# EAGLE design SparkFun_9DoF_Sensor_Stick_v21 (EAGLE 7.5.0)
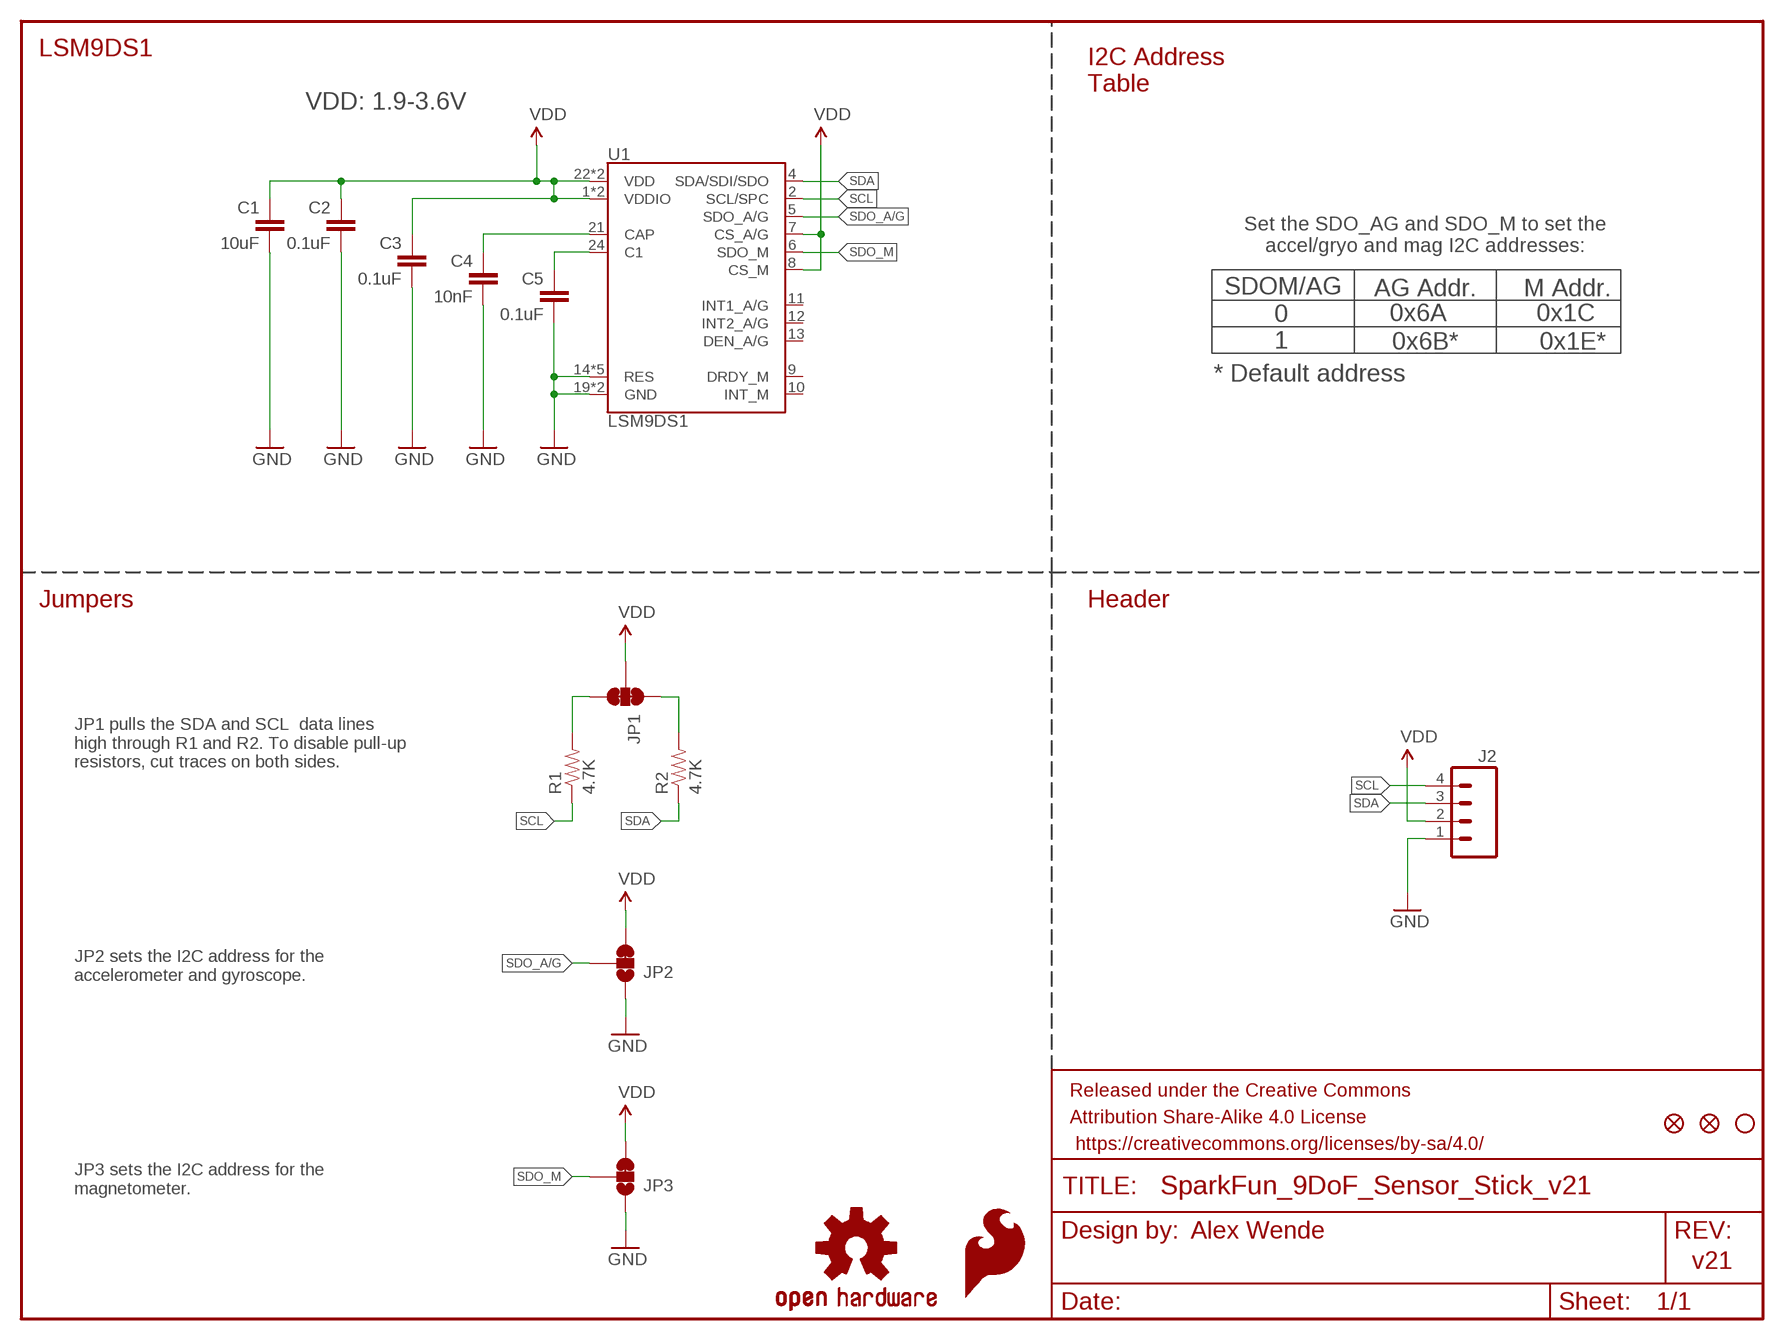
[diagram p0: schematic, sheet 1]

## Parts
C1  10uF  10UF-6.3V-20%(0603)  [0603-CAP]
C2  0.1uF  0.1UF-25V(+80/-20%)(0603)  [0603-CAP]
C3  0.1uF  0.1UF-25V(+80/-20%)(0603)  [0603-CAP]
C4  10nF  10NF/10000PF-50V-10%(0603)  [0603-CAP]
C5  0.1uF  0.1UF-25V(+80/-20%)(0603)  [0603-CAP]
FD3  FIDUCIALUFIDUCIAL  [MICRO-FIDUCIAL]
FD4  FIDUCIALUFIDUCIAL  [MICRO-FIDUCIAL]
FRAME1  FRAME-LETTER  [CREATIVE_COMMONS]
H1  STAND-OFF  [STAND-OFF]
J2  M04NO_SILK_ALL_ROUND  [1X04_NO_SILK_ALL_ROUND]
JP1  JUMPER-PAD-3-NC_BY_TRACE  [PAD-JUMPER-3-3OF3_NC_BY_TRACE_YES_SILK_FULL_BOX]
JP2  JUMPER-PAD-3-2OF3_NC_BY_TRACE_SMALL  [PAD-JUMPER-3-2OF3_NC_BY_TRACE_YES_SILK_FULL_BOX]
JP3  JUMPER-PAD-3-2OF3_NC_BY_TRACE_SMALL  [PAD-JUMPER-3-2OF3_NC_BY_TRACE_YES_SILK_FULL_BOX]
LOGO1  SFE_LOGO_FLAME.1_INCH  [SFE_LOGO_FLAME_.1]
LOGO3  OSHW-LOGOMINI  [OSHW-LOGO-MINI]
R1  4.7K  4.7KOHM-1/10W-1%(0603)  [0603-RES]
R2  4.7K  4.7KOHM-1/10W-1%(0603)  [0603-RES]
U1  LSM9DS1  [LGA24-8X4]

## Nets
GND: C1.2 C2.2 C3.2 C4.2 C5.2 J2.1 JP2.1 JP3.1 U1.14(RES) U1.15(RES) U1.16(RES) U1.17(RES) U1.18(RES) U1.19(GND) U1.20(GND)
N$1: JP1.1 R2.2
N$2: JP1.3 R1.2
N$5: C4.1 U1.21(CAP)
N$6: C5.1 U1.24(C1)
SCL: J2.4 R1.1 U1.2(SCL/SPC)
SDA: J2.3 R2.1 U1.4(SDA/SDI/SDO)
SDO_A/G: JP2.2 U1.5(SDO_A/G)
SDO_M: JP3.2 U1.6(SDO_M)
VDD: C1.1 C2.1 C3.1 J2.2 JP1.2 JP2.3 JP3.3 U1.1(VDDIO) U1.3(VDDIO) U1.7(CS_A/G) U1.8(CS_M) U1.22(VDD) U1.23(VDD)
Unconnected: U1.9(DRDY_M) U1.10(INT_M) U1.11(INT1_A/G) U1.12(INT2_A/G) U1.13(DEN_A/G)

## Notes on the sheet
- LSM9DS1
- I2C Address
  Table
- VDD: 1.9-3.6V
- Set the SDO_AG and SDO_M to set the
  accel/gryo and mag I2C addresses:
- SDOM/AG | AG Addr. | M Addr.
- 0x6A | 0x1C
- 0
  1
- 0x6B* | 0x1E*
- * Default address
- Jumpers | Header
- JP1 pulls the SDA and SCL  data lines
  high through R1 and R2. To disable pull-up
  resistors, cut traces on both sides.
- JP2 sets the I2C address for the
  accelerometer and gyroscope.
- JP3 sets the I2C address for the
  magnetometer.
- Alex Wende
- v21

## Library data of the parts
C1 = SparkFun-Capacitors:10UF-6.3V-20%(0603): CAP-11015; PROD_ID: CAP-11015
C2 C3 C5 = SparkFun-Capacitors:0.1UF-25V(+80/-20%)(0603): CAP-00810; PROD_ID: CAP-00810
C4 = SparkFun-Capacitors:10NF/10000PF-50V-10%(0603): CAP-00867; PROD_ID: CAP-00867
FD3 FD4 = SparkFun-Aesthetics:FIDUCIAL: Fiducial Alignment Points
FRAME1 = SparkFun-Aesthetics:FRAME-LETTER: Schematic Frame
H1 = SparkFun-Electromechanical:STAND-OFF: #4 Stand Off
J2 = SparkFun-Connectors:M04: Header 4 Standard 4-pin 0.1" header. Use with straight break away headers (SKU : PRT-00116), right angle break away headers (PRT-00553), swiss pins (PRT-00743), machine pins (PRT-00117), and female headers (PRT-00115). Molex polarized connector foot print use with SKU : PRT-08231 with associated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; PROD_ID: CONN-09696
JP1 = SparkFun-Passives:JUMPER-PAD-3-NC_BY_TRACE
JP2 JP3 = SparkFun-Passives:JUMPER-PAD-3-2OF3_NC_BY_TRACE
LOGO1 = SparkFun-Aesthetics:SFE_LOGO_FLAME: SFE Logo, flame only
LOGO3 = SparkFun-Aesthetics:OSHW-LOGO: Open Source Hardware Logo
R1 R2 = SparkFun-Resistors:4.7KOHM-1/10W-1%(0603): RES-07857; PROD_ID: RES-07857
U1 = SparkFun-Sensors:LSM9DS1: LSM9DS1 3D accelerometer, gyroscope & magnetometer The LSM9DS1 is a system-in-package featuring a 3D digital linear acceleration sensor, a 3D digital angular rate sensor, and a 3D digital magnetic sensor. The LSM9DS1 has a linear acceleration full scale of ±2g/±4g/±8/±16 g, a magnetic field full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; PROD_ID: IC-12536

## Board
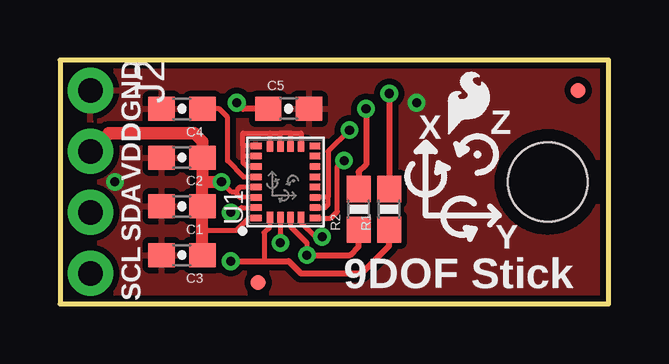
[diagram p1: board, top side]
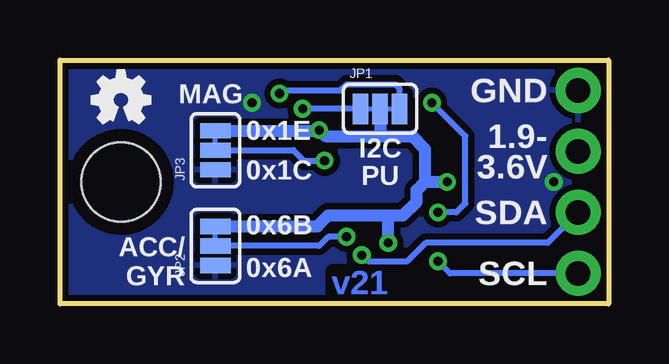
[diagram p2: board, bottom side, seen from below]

Size 22.86 x 10.16 mm. Coordinates in mm from the lower left corner, seen from the top.
Outline: 0,0 22.86,0 22.86,10.16 0,10.16 0,0
Copper layers (1*16): Top 0.035mm / dielectric 1.5mm / Bottom 0.035mm
Design rules "SparkFun-2-layer-TIGHT": minimum track width 7mil, minimum drill 15mil, track to track 7mil, track to pad 7mil, pad to pad 7mil, via to via 7mil, smd to smd 7mil, copper to edge 7mil, drill to drill 7mil, minimum pad ring 7mil, minimum via ring 7mil, stop-mask expansion 4mil, vias tented up to drill 25mil, thermal gap 10mil

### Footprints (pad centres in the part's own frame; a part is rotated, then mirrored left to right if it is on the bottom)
0603-CAP = smd 1.1 x 1: 1 -0.85,0; 2 0.85,0
MICRO-FIDUCIAL = smd 0.635 x 0.635: 1 0,0
STAND-OFF = hole 3.302: 0,0
1X04_NO_SILK_ALL_ROUND = drill 1.016 pad 1.88: 1 0,0; 2 2.54,0; 3 5.08,0; 4 7.62,0
PAD-JUMPER-3-3OF3_NC_BY_TRACE_YES_SILK_FULL_BOX = smd 0.635 x 1.27: 1 -0.813,0; 2 0,0; 3 0.813,0
PAD-JUMPER-3-2OF3_NC_BY_TRACE_YES_SILK_FULL_BOX = smd 0.635 x 1.27: 1 -0.813,0; 2 0,0; 3 0.813,0
0603-RES = smd 1.1 x 1: 1 -0.85,0; 2 0.85,0
LGA24-8X4 = smd 0.27 x 0.45: 1 -1.505,1.225; 6 -1.505,-1.225; 7 -1.075,-1.225; 8 -0.645,-1.225; 9 -0.215,-1.225; 10 0.215,-1.225; 11 0.645,-1.225; 12 1.075,-1.225; 13 1.505,-1.225; 18 1.505,1.225; 19 1.075,1.225; 20 0.645,1.225; 21 0.215,1.225; 22 -0.215,1.225; 23 -0.645,1.225; 24 -1.075,1.225 | smd 0.45 x 0.27: 2 -1.475,0.645; 3 -1.475,0.215; 4 -1.475,-0.215; 5 -1.475,-0.645; 14 1.475,-0.645; 15 1.475,-0.215; 16 1.475,0.215; 17 1.475,0.645

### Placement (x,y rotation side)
C1  5.08,4.06 180 top
C2  5.08,6.1 180 top
C3  5.08,2.03 180 top
C4  5.08,8.13 180 top
C5  9.53,8.13 0 top
FD3  8.26,0.89 0 top
FD4  21.59,8.89 0 top
FRAME1  not placed on the board
H1  20.32,5.08 0 top
J2  1.27,8.89 270 top
JP1  9.53,8.13 0 bottom
JP2  16.38,2.41 90 bottom
JP3  16.38,6.4 90 bottom
LOGO1  15.88,6.73 0 top
LOGO3  20.32,8.51 0 bottom
R1  13.72,3.94 90 top
R2  12.45,3.94 90 top
U1  9.4,5.08 90 top

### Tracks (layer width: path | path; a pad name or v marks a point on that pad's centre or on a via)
GND  (via drill 0.38)
  Top 0.203: 7.84,5.72 U1.20 7.79,5.72 7.62,5.9 7.62,6.16 | 7.62,6.58 7.62,7.11 8.75,7.11 | 9.61,7.11 10.04,7.11 U1.14 | U1.19 7.62,6.16 | U1.18 7.62,6.58 | 7.62,6.58 7.62,6.16 | U1.17 8.75,7.11 | U1.16 9.18,7.11 | U1.15 9.61,7.11 | 9.61,7.11 9.18,7.11 | 8.75,7.11 9.18,7.11
  other vias: 2.29,5.08 14.86,8.38
  pour Top (isolate 0.254): 0,10.16 0,0 22.86,0 22.86,10.16
  pour Bottom (isolate 0.254): 0,10.16 0,0 22.86,0 22.86,10.16
N$1  (via drill 0.38)
  Top 0.254: v12.75,8.13 12.75,5.8 12.45,5.5 R2.2
  Bottom 0.254: JP1.1 v12.75,8.13
N$2  (via drill 0.38)
  Top 0.254: v13.72,8.76 R1.2
  Bottom 0.254: JP1.3 8.71,8.97 8.89,9.14 10.92,9.14 11.18,8.89 13.72,8.89 v13.72,8.76
N$5
  Top 0.203: U1.21 7.64,5.29 6.99,5.95 6.99,7.77 6.63,8.13 C4.1
N$6  (via drill 0.38)
  Top 0.203: v7.11,3.81 7.37,3.81 7.56,4 U1.24
  Top 0.254: C5.1 7.62,8.13 v7.37,8.38
  Bottom 0.254: v7.37,8.38 5.97,6.99 5.97,4.19 6.35,3.81 v7.11,3.81
SCL  (via drill 0.38)
  Top 0.203: U1.2 8.75,3.22 8.51,2.98 8.51,1.78
  Top 0.254: R1.1 13.72,2.41 12.57,1.27 12.32,1.27 10.03,1.27 9.53,1.78 8.51,1.78 v7.11,1.78
  Bottom 0.254: J2.4 6.6,1.27 v7.11,1.78
SDA  (via drill 0.38)
  Top 0.203: U1.4 9.61,3.21 10.29,2.54 v10.29,2.03
  Top 0.254: v10.29,2.03 12.09,2.03 12.45,2.39 R2.1
  Bottom 0.254: J2.3 2.54,2.54 7.62,2.54 8.38,1.78 10.03,1.78 v10.29,2.03
SDO_A/G  (via drill 0.38)
  Top 0.203: U1.5 10.04,3.42 10.03,3.41 10.65,2.79 v10.92,2.79 10.67,2.79
  Bottom 0.254: v10.92,2.79 11.68,2.79 12.06,2.41 JP2.2
SDO_M  (via drill 0.38)
  Top 0.203: U1.6 11.29,3.58 11.56,3.85 11.56,5.71 11.84,5.99 v11.84,5.97
  Bottom 0.254: v11.84,5.97 12.7,5.97 13.13,6.4 JP3.2
VDD  (via drill 0.38)
  Top 0.203: U1.22 7.5,4.87 7.37,4.73 7.37,4.65 | U1.23 7.49,4.43 7.37,4.56 7.37,4.65 | 7.37,4.65 7.16,4.65 v6.73,5.08 | U1.1 7.87,3.58 7.35,3.05 5.93,3.05 | U1.7 11.04,4 11.18,4.14 11.18,4.43 | v12.06,7.24 11.18,6.35 11.18,4.43 | 11.18,4.43 U1.8 | U1.3 v9.18,2.54
  Top 0.508: 5.93,5.08 C2.1 5.93,6.77 5.59,7.11 | C3.1 5.93,3.05 C1.1 5.93,5.08 | 5.93,5.08 v6.73,5.08 | J2.2 2.03,7.11
  Top 0.516: 2.03,7.11 5.59,7.11
  Bottom 0.508: JP1.2 9.53,6.99 | 9.53,6.99 8.19,6.99 7.66,6.45 7.66,5.08 | 7.66,5.08 v6.73,5.08 | 7.66,5.08 8,4.74 8,4.25 8.57,3.68 9.18,3.68 | 9.53,6.99 11.81,6.99 v12.06,7.24 12.09,7.21 JP3.3 | 9.18,3.68 11.68,3.68 12.14,3.23 JP2.3 | v9.18,2.54 9.18,3.68

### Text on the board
Bottom: v21
tPlace: GND | X | Z | VDD | SDA | Y | SCL | 9DOF Stick
bPlace: GND | MAG | 1.9- | 0x1E | 3.6V | I2C | 0x1C | PU | SDA | 0x6B | 0x6A | ACC/ / GYR | SCL
Measures: Units are in Inches
tDocu: PCB thickness = 0.032" | Alex Wende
